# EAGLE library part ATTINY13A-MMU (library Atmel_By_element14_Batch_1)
Microcontroller
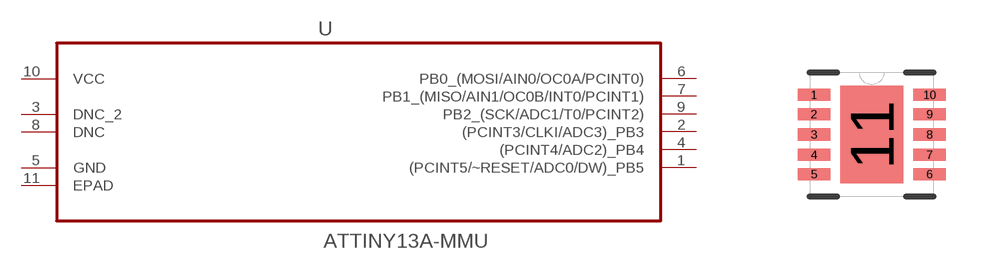
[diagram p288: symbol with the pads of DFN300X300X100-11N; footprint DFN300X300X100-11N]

Designator prefix U

## ATTINY13A-MMU (DESCRIPTION: Microcontroller; MPN: ATTINY13A-MMU; OC_FARNELL: 1715516; OC_NEWARK: 15R0298; PACKAGE: DFN-10; SUPPLIER: ATMEL)  [DFN300X300X100-11N]
1  (PCINT5/~RESET/ADC0/DW)_PB5
2  (PCINT3/CLKI/ADC3)_PB3
3  DNC_2  nc
4  (PCINT4/ADC2)_PB4
5  GND  pas
6  PB0_(MOSI/AIN0/OC0A/PCINT0)
7  PB1_(MISO/AIN1/OC0B/INT0/PCINT1)
8  DNC  nc
9  PB2_(SCK/ADC1/T0/PCINT2)
10  VCC  pwr
11  EPAD  pas

## Footprint DFN300X300X100-11N (pad centres in mm)
smd 0.813 x 0.305: 1 -1.448,0.991; 2 -1.448,0.508; 3 -1.448,0; 4 -1.448,-0.508; 5 -1.448,-0.991; 6 1.448,-0.991; 7 1.448,-0.508; 8 1.448,0; 9 1.448,0.508; 10 1.448,0.991
smd 1.575 x 2.438: 11 0,0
